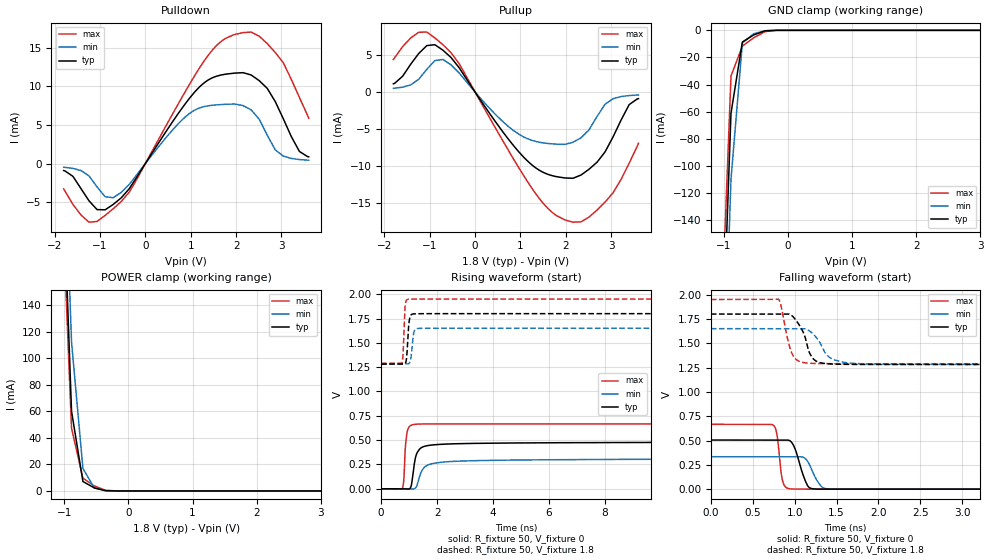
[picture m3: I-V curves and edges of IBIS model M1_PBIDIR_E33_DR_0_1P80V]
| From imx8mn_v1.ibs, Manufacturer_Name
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[Model] M1_PBIDIR_E33_DR_0_1P80V
Model_type I/O
Vinl  =  0.54
Vinh  =  1.26
Vmeas =  0.9
| Capacitance   typ   min   max
C_comp   8.99140471561e-13   8.21462742958e-13   9.40633374847e-13
| Variables   typ   min   max
[GND Clamp Reference]   0   0   0
[POWER Clamp Reference]   1.8   1.65   1.95
[Pulldown Reference]   0   0   0
[Pullup Reference]   1.8   1.65   1.95
[Temperature Range]   25   125   -40
[Voltage Range]   1.8   1.65   1.95
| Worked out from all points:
|   slope of the pulldown table from 0 to 0.27 V, typ, clamps not added: 109 ohm
|   slope of the pullup table from 0 to 0.27 V, typ, clamps not added: 110 ohm
|   GND clamp passes 1 mA (typ) near -0.39 V on its own axis
|   POWER clamp passes 1 mA (typ) near -0.43 V on its own axis
|   falling waveform, R_fixture 50, V_fixture 0: 20-80 % time 111ps typ, 115ps min, 51.1ps max; typ from 0.505 V to 0 V
|   falling waveform, R_fixture 50, V_fixture 1.8: 20-80 % time 139ps typ, 174ps min, 101ps max; typ from 1.8 V to 1.28 V
|   rising waveform, R_fixture 50, V_fixture 0: 20-80 % time 224ps typ, 536ps min, 82.2ps max; typ from 0 V to 0.492 V
|   rising waveform, R_fixture 50, V_fixture 1.8: 20-80 % time 69.7ps typ, 78.1ps min, 51.4ps max; typ from 1.28 V to 1.8 V
[GND Clamp]
| Voltage   I(typ)   I(min)   I(max)
-1.8V     -1.562A    -1.614A    -1.516A
-1.064V   -296mA     -355.2mA   -250.4mA
-886.4mV  -61.18mA   -109.9mA   -33.74mA
-709.1mV  -8.602mA   -9.384mA   -11.67mA
-531.8mV  -3.4mA     -2.481mA   -5.473mA
-354.5mV  -361.2uA   -272.6uA   -975.8uA
-177.3mV  -1.362uA   -3.436uA   -2.724uA
3.6V      0A         0A         0A
[POWER Clamp]
| Voltage   I(typ)   I(min)   I(max)
-1.8V     1.563A     1.607A     1.521A
-1.064V   296.1mA    350.6mA    257.7mA
-886.4mV  60.03mA    112.2mA    47.22mA
-709.1mV  7.094mA    16.96mA    9.663mA
-531.8mV  2.299mA    2.209mA    3.776mA
-354.5mV  136.5uA    326.9uA    430.1uA
-177.3mV  338.8nA    11.95uA    535.8nA
3.6V      0A         0A         0A
[Pulldown]
| Voltage   I(typ)   I(min)   I(max)
-1.8V     -907.9uA   -480.6uA   -3.27mA
-1.241V   -4.822mA   -1.6mA     -7.583mA
-1.064V   -5.953mA   -3.021mA   -7.483mA
-709.1mV  -5.289mA   -4.421mA   -5.854mA
-354.5mV  -3.257mA   -2.701mA   -3.696mA
956.3mV   8.318mA    6.398mA    10.09mA
1.519V    11.19mA    7.562mA    14.95mA
1.977V    11.7mA     7.693mA    16.7mA
2.332V    11.45mA    6.945mA    17mA
2.864V    8.001mA    1.765mA    14.36mA
3.395V    1.564mA    518.9uA    8.539mA
3.6V      868.9uA    436.5uA    5.864mA
[Pullup]
| Voltage   I(typ)   I(min)   I(max)
-1.8V     1.123mA    505.2uA    4.414mA
-1.241V   5.233mA    1.734mA    8.115mA
-886.4mV  6.422mA    4.267mA    7.345mA
-354.5mV  3.331mA    2.605mA    3.881mA
506.2mV   -4.515mA   -3.386mA   -5.491mA
1.097V    -9.001mA   -6.169mA   -11.59mA
1.575V    -11.1mA    -6.962mA   -15.6mA
1.977V    -11.66mA   -7.099mA   -17.34mA
2.509V    -10.49mA   -5.15mA    -16.97mA
2.864V    -8.13mA    -1.661mA   -14.94mA
3.395V    -1.708mA   -477.2uA   -9.663mA
3.6V      -899.4uA   -397.7uA   -6.967mA
[Ramp]
dV/dt_r   0.295342/0.224144n  0.194516/0.53575n  0.399949/82.1832p
dV/dt_f   0.311098/0.138924n  0.220378/0.173511n  0.396442/0.101357n
R_load = 50
[Falling Waveform]
R_fixture = 50
V_fixture = 0
V_fixture_min = 0
V_fixture_max = 0
| Time   V(typ)   V(min)   V(max)
0s        505mV      333.7mV    666.6mV
745.2ps   505mV      333.7mV    657.3mV
786.9ps   504.9mV    333.7mV    571.8mV
838.4ps   505.2mV    333.7mV    170.9mV
870.2ps   505.3mV    333.7mV    48.99mV
987.7ps   448.1mV    333.9mV    1.415mV
1.144ns   52.7mV     299.4mV    298uV
1.34ns    434.6uV    14.55mV    98.54uV
1.743ns   83.7uV     226.9uV    39.26uV
333.3ns   251.3nV    1.176uV    236.6nV
[Falling Waveform]
R_fixture = 50
V_fixture = 1.8
V_fixture_min = 1.65
V_fixture_max = 1.95
| Time   V(typ)   V(min)   V(max)
0s        1.8V       1.65V      1.95V
803.8ps   1.8V       1.65V      1.953V
836.8ps   1.8V       1.65V      1.886V
938.9ps   1.799V     1.65V      1.467V
1.008ns   1.745V     1.65V      1.341V
1.106ns   1.607V     1.65V      1.301V
1.225ns   1.337V     1.591V     1.292V
1.392ns   1.289V     1.373V     1.29V
1.553ns   1.284V     1.31V      1.289V
333.3ns   1.282V     1.283V     1.289V
[Rising Waveform]
R_fixture = 50
V_fixture = 0
V_fixture_min = 0
V_fixture_max = 0
| Time   V(typ)   V(min)   V(max)
0s        154.7nV    1.146uV    177nV
755.6ps   -66.11uV   222.4nV    -114.5uV
812.2ps   -114.3uV   153.1nV    96.18mV
871.9ps   -1.175mV   -48.55uV   449.3mV
950.9ps   -3.663mV   -141.3uV   606.3mV
1.076ns   30.44mV    -1.861mV   653.3mV
1.262ns   354.5mV    20.66mV    664mV
1.536ns   435mV      217.6mV    666.3mV
19.73ns   480.4mV    308.8mV    666.6mV
333.3ns   492.2mV    324.2mV    666.6mV
[Rising Waveform]
R_fixture = 50
V_fixture = 1.8
V_fixture_min = 1.65
V_fixture_max = 1.95
| Time   V(typ)   V(min)   V(max)
0s        1.282V     1.283V     1.289V
747.6ps   1.281V     1.283V     1.297V
783.6ps   1.281V     1.283V     1.381V
836.2ps   1.283V     1.283V     1.786V
873.7ps   1.294V     1.283V     1.912V
1.003ns   1.723V     1.29V      1.949V
1.139ns   1.797V     1.552V     1.95V
1.244ns   1.799V     1.643V     1.95V
1.965ns   1.8V       1.65V      1.95V
333.3ns   1.8V       1.65V      1.95V
[Add Submodel]
| Submodel Name Mode
M1_PBIDIR_E33_DR_0_1P80V_T All
